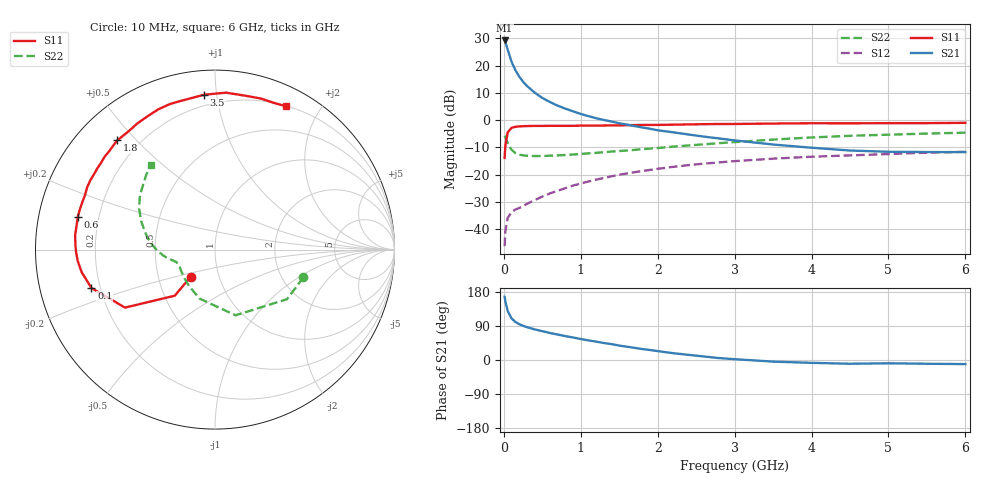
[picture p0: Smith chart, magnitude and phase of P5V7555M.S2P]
! SIEMENS Small Signal Semiconductors
! BFP183
! Si NPN RF Bipolar Junction Transistor in SOT143
! VCE = 0.75 V  IC = 55 mA
! Common Emitter S-Parameters:  March  1996
# GHz  S  MA  R  50
!  f  S11  S21  S12  S22
! GHz  MAG  ANG  MAG  ANG  MAG  ANG  MAG  ANG
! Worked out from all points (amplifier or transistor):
!   36 points, 10 MHz to 6 GHz, reference 50 ohm
!   highest |S21| = 29.2 dB at 10 MHz (marker M1)
!   |S21| within 3 dB of that: start of sweep to 46.14 MHz
!   unconditionally stable (mu >= 1): start of sweep to 37.21 MHz; 119 MHz to end of sweep
!   at 250 MHz: K = 1.50, MAG = 18.6 dB, |S12| = -31.5 dB
!   at 1.4 GHz: K = 2.08, MAG = 4.1 dB, |S12| = -20.6 dB
!   at 6 GHz: K = 1.52, MAG = -4.3 dB, |S12| = -11.6 dB
!   S11 on the Smith chart (normalised r, x): 10 MHz: 0.73, -0.23; 100 MHz: 0.17, -0.15; 600 MHz: 0.12, +0.12; 1.8 GHz: 0.12, +0.44; 3.5 GHz: 0.13, +0.92; 6 GHz: 0.21, +1.59
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0.01  0.2034 -131.8  28.81 167.0  0.0049 60.8  0.5164 -17.4
0.02  0.3408 -131.1  27.13 154.9  0.0092 59.6  0.4873 -34.5
0.05  0.5965 -147.2  19.56 129.2  0.0162 46.9  0.3836 -72.6
0.1  0.7207 -162.7  11.77 109.8  0.0205 37.4  0.2863 -107.4
0.15  0.7536 -170.4  8.239 100.5  0.023 38.4  0.2491 -125.7
0.2  0.7673 -175.2  6.269 94.6  0.0245 40.2  0.2335 -136.5
0.25  0.774 -178.9  5.052 90.2  0.0265 42.2  0.226 -143.5
0.3  0.7778 178.3  4.231 86.7  0.0292 45.6  0.2222 -148.4
0.4  0.7835 174.1  3.194 80.9  0.0342 50.9  0.2195 -154.2
0.5  0.7827 169.8  2.548 76.0  0.0397 53.3  0.2201 -157.8
0.6  0.7864 166.5  2.146 71.3  0.0454 55.8  0.2229 -160.2
0.7  0.7854 163.1  1.837 67.1  0.0508 56.9  0.2258 -162.0
0.8  0.785 160.0  1.62 63.1  0.0567 58.0  0.2295 -162.9
1.1  0.7944 151.0  1.182 51.7  0.0752 57.6  0.246 -166.2
1.5  0.8037 140.0  0.876 38.0  0.0999 54.9  0.2713 -170.4
1.8  0.8163 131.8  0.733 28.9  0.1167 51.8  0.2938 -174.0
2.2  0.8252 121.7  0.598 18.0  0.139 46.8  0.3264 180.0
2.8  0.8489 107.4  0.461 5.0  0.1683 38.7  0.3784 170.5
3.5  0.865 94.0  0.357 -4.3  0.1966 29.9  0.4395 159.2
4.5  0.8738 79.0  0.277 -9.9  0.2259 18.0  0.5163 144.1
5.5  0.8806 68.2  0.26 -9.9  0.2535 8.0  0.567 132.4
6  0.8909 63.7  0.259 -10.8  0.2624 2.7  0.5884 127.1
